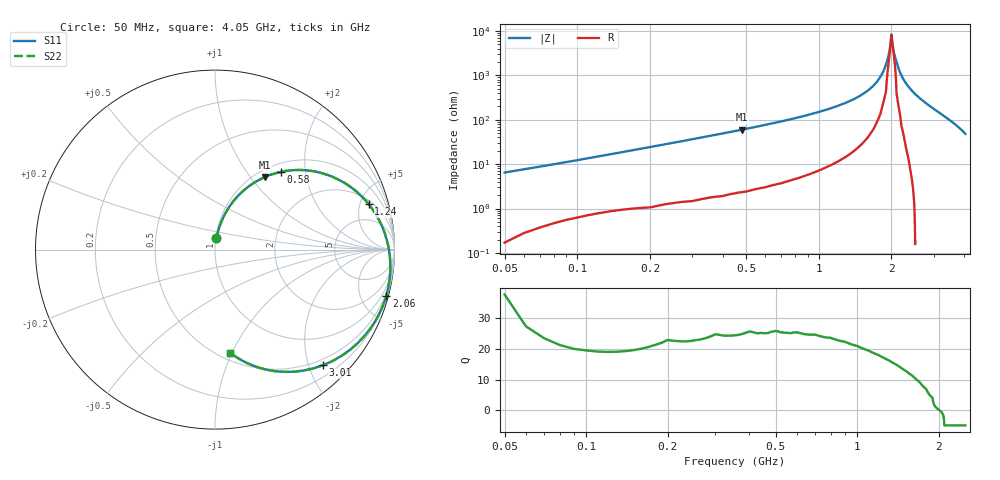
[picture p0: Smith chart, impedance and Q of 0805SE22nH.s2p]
! AVX Thin Film Operation		Date: May 2002
! Description: Accu-L® Series, Thin Film, SMD, RF Inductors
! Part Number: L0805220GEWTR
! 50 MHz  -  4.05 GHz
! Serial Measurements
# mhz S db R 50
!	S11		S21		S12		S22
!	dB	Phase	dB	Phase	dB	Phase	dB	Phase
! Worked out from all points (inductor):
!   401 points, 50 MHz to 4.05 GHz, reference 50 ohm
!   read as one part in series: L = 19.5 nH near 70 MHz
!   highest Q = 25.5 at 480 MHz (marker M1), where L = 19.8 nH
!   self-resonance near 2.014 GHz
!   S11 on the Smith chart (normalised r, x): 50 MHz: 1.01, +0.13; 580 MHz: 1.15, +1.48; 1.24 GHz: 2.39, +5.97; 2.06 GHz: 0.35, -7.52; 3.01 GHz: 0.39, -2.24; 4.05 GHz: 0.57, -0.98
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50  -24.07 82.9  -0.01 -3.8  -0.01 -3.8  -24.07 82.9
120  -17.17 78.3  -0.15 -8.6  -0.15 -8.6  -17.17 78.3
200  -12.94 73.2  -0.31 -14.1  -0.31 -14.1  -12.94 73.2
480  -6.19 55.5  -1.37 -32.0  -1.37 -32.0  -6.19 55.5
580  -4.89 49.6  -1.91 -37.9  -1.91 -37.9  -4.89 49.6
720  -3.54 41.7  -2.80 -45.7  -2.80 -45.7  -3.54 41.7
1240  -0.99 16.5  -7.62 -70.0  -7.62 -70.0  -0.99 16.5
1390  -0.64 10.1  -9.65 -75.9  -9.65 -75.9  -0.64 10.1
1630  -0.29 0.6  -14.16 -83.9  -14.20 -83.9  -0.29 0.6
1800  -0.15 -5.8  -19.52 -87.4  -19.50 -87.4  -0.15 -5.8
1920  -0.11 -10.1  -26.73 -73.2  -26.70 -73.2  -0.11 -10.1
2000  -0.10 -13.0  -38.67 -25.3  -38.70 -25.3  -0.10 -13.0
2020  -0.10 -13.7  -34.48 -7.8  -34.50 -7.8  -0.10 -13.7
2050  -0.10 -14.8  -30.54 18.5  -30.50 18.5  -0.10 -14.8
2060  -0.10 -15.1  -29.54 27.3  -29.50 27.3  -0.10 -15.1
2160  -0.12 -18.6  -22.34 64.4  -22.30 64.4  -0.12 -18.6
2280  -0.17 -22.7  -17.51 65.0  -17.50 65.0  -0.17 -22.7
2470  -0.32 -29.1  -13.13 60.7  -13.10 60.7  -0.32 -29.1
2720  -0.61 -37.5  -9.62 53.6  -9.62 53.6  -0.61 -37.5
3010  -1.10 -47.1  -6.93 44.9  -6.93 44.9  -1.10 -47.1
3390  -2.05 -59.6  -4.54 33.2  -4.54 33.2  -2.05 -59.6
4050  -4.73 -81.7  -1.98 12.5  -1.98 12.5  -4.73 -81.7
